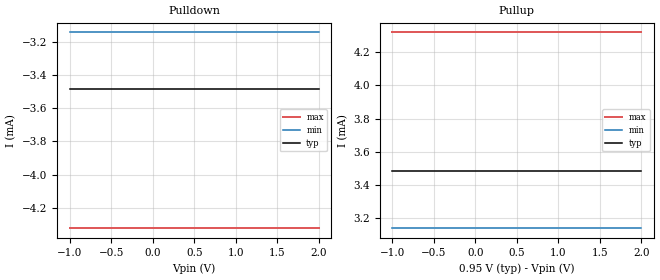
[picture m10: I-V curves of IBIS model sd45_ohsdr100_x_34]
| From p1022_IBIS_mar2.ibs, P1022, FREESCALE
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[Model]   sd45_ohsdr100_x_34
Model_type 3-state
Enable Active-High
Polarity Non-Inverting
|   TYP   MIN   MAX
C_comp   0.00pF   0.00pF   0.00pF
[Model Spec]
Vmeas   0.475   0.425   0.605
[Temperature Range] 65   125   -40
[Voltage Range]   0.95   0.85   1.21
[Pullup]
|   Vout(V)   TYP   WCS   BCS
-1V       3.486mA    3.14mA     4.319mA
2V        3.486mA    3.14mA     4.319mA
[Pulldown]
|   Vout(V)   TYP   WCS   BCS
-1V       -3.486mA   -3.142mA   -4.323mA
2V        -3.486mA   -3.142mA   -4.323mA
[GND Clamp]
|   Vout(V)   TYP   WCS   BCS
-1V       0A         0A         0A
1V        0A         0A         0A
[POWER Clamp]
|   Vout(V)   TYP   WCS   BCS
-1V       0A         0A         0A
0V        0A         0A         0A
[Ramp]
R_load=50
dV/dt_r  2.2428e-01/6.4141e-11  1.9173e-01/6.5657e-11  3.0370e-01/6.5055e-11
dV/dt_f  2.2428e-01/6.6042e-11  1.9173e-01/6.8481e-11  3.0372e-01/6.6195e-11
|[End   sd45_ohsdr100_x_34
